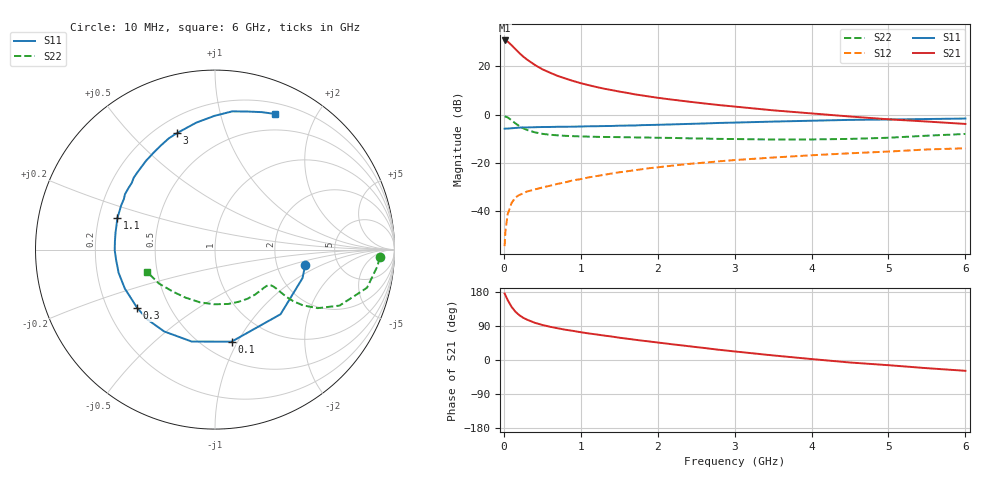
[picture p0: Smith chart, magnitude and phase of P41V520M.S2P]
! SIEMENS Small Signal Semiconductors
! BFP182
! Si NPN RF Bipolar Junction Transistor in SOT143
! VCE = 1.5 V  IC = 20 mA
! Common Emitter S-Parameters:  March  1996
# GHz  S  MA  R  50
!  f  S11  S21  S12  S22
! GHz  MAG  ANG  MAG  ANG  MAG  ANG  MAG  ANG
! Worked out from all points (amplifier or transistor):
!   36 points, 10 MHz to 6 GHz, reference 50 ohm
!   highest |S21| = 30.6 dB at 10 MHz (marker M1)
!   |S21| within 3 dB of that: start of sweep to 132.7 MHz
!   unconditionally stable (mu >= 1): 487.2 MHz to end of sweep
!   at 250 MHz: K = 0.64, MSG = 28.3 dB, |S12| = -32.6 dB
!   at 1.4 GHz: K = 1.41, MAG = 13.5 dB, |S12| = -24.4 dB
!   at 6 GHz: K = 1.06, MAG = 3.5 dB, |S12| = -13.9 dB
!   S11 on the Smith chart (normalised r, x): 10 MHz: 2.92, -0.66; 100 MHz: 0.67, -0.94; 300 MHz: 0.33, -0.30; 1.1 GHz: 0.28, +0.15; 3 GHz: 0.28, +0.68; 6 GHz: 0.31, +1.49
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0.01  0.5101 -9.4  34.04 175.5  0.0019 78.2  0.9189 -2.7
0.02  0.5127 -18.1  34.02 171.3  0.0038 82.1  0.9098 -5.8
0.05  0.5129 -44.6  32.28 158.1  0.0087 73.7  0.8732 -14.1
0.1  0.5212 -79.8  27.22 140.4  0.0148 59.7  0.761 -24.2
0.15  0.5285 -104.2  22.59 127.6  0.0193 52.9  0.6584 -29.7
0.2  0.5367 -121.8  18.82 118.4  0.0217 49.1  0.5793 -32.4
0.25  0.5418 -134.1  15.88 111.6  0.0234 47.4  0.5212 -33.4
0.3  0.5416 -143.2  13.78 106.6  0.0256 46.2  0.4814 -33.5
0.4  0.5472 -156.6  10.7 98.4  0.0282 46.2  0.4303 -32.9
0.5  0.5524 -166.5  8.651 92.5  0.031 47.1  0.3997 -32.4
0.6  0.5539 -174.0  7.339 87.7  0.0338 49.3  0.3825 -32.3
0.7  0.5587 -179.6  6.291 83.7  0.0369 50.6  0.3715 -32.5
0.8  0.5594 175.4  5.564 79.9  0.0398 51.6  0.3633 -33.1
1  0.5659 165.7  4.448 73.3  0.0462 53.2  0.3529 -34.9
1.1  0.5721 161.8  4.064 70.2  0.0501 53.1  0.3495 -36.2
1.5  0.5887 148.5  2.99 58.9  0.064 53.4  0.3413 -42.3
2.2  0.6266 127.8  2.023 41.2  0.0882 49.4  0.3285 -56.4
3  0.6823 108.3  1.463 22.6  0.1145 43.1  0.3117 -76.4
3.5  0.7154 98.3  1.223 12.1  0.1293 38.7  0.3047 -90.9
4.5  0.7761 82.9  0.911 -6.6  0.1581 30.0  0.3138 -121.4
5.5  0.8086 71.3  0.717 -21.6  0.1895 21.2  0.3656 -149.0
6  0.8268 66.1  0.64 -28.5  0.2011 15.9  0.397 -161.5
